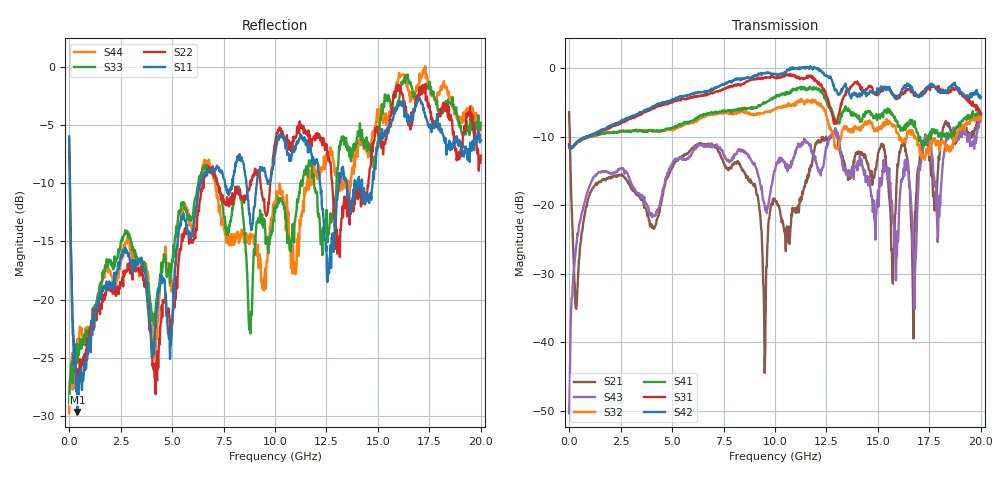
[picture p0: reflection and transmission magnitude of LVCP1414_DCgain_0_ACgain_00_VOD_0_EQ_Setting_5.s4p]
!Agilent Technologies,N5230A,MY46400459,A.07.50.48
!Agilent N5230A: A.07.50.48
!Date: Tuesday, April 17, 2012 18:35:00
!Correction: S11(Full 4 Port(1,2,3,4))
!S12(Full 4 Port(1,2,3,4))
!S13(Full 4 Port(1,2,3,4))
!S14(Full 4 Port(1,2,3,4))
!S21(Full 4 Port(1,2,3,4))
!S22(Full 4 Port(1,2,3,4))
!S23(Full 4 Port(1,2,3,4))
!S24(Full 4 Port(1,2,3,4))
!S31(Full 4 Port(1,2,3,4))
!S32(Full 4 Port(1,2,3,4))
!S33(Full 4 Port(1,2,3,4))
!S34(Full 4 Port(1,2,3,4))
!S41(Full 4 Port(1,2,3,4))
!S42(Full 4 Port(1,2,3,4))
!S43(Full 4 Port(1,2,3,4))
!S44(Full 4 Port(1,2,3,4))
!S4P File: Measurements: <S11,S12,S13,S14>,
!<S21,S22,S23,S24>,
!<S31,S32,S33,S34>,
!<S41,S42,S43,S44>:
# Hz S  dB  R 50
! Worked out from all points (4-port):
!   801 points, 300 kHz to 20 GHz, reference 50 ohm
!   strongest paths, dB at 300 kHz, 5 GHz, 10 GHz, 15 GHz, 20 GHz:
!     S42: -11.4, -4.5, -0.8, -3.1, -4.2
!     S31: -11.1, -5.0, -1.4, -3.9, -6.6
!     S41: -11.2, -8.6, -4.3, -7.1, -6.6
!     S32: -11.3, -9.0, -6.0, -9.0, -7.4
!     S43: -50.4, -13.9, -15.0, -17.8, -7.5
!     S21: -6.4, -14.5, -19.2, -12.4, -7.0
!   lowest |S11| = -29.7 dB at 400.3 MHz (marker M1), VSWR 1.07, Z = 53.1 + j1.45 ohm
!   |S11| at or under -10 dB: 37.44 MHz to 6.372 GHz (6.335 GHz wide, 198 % of centre); 8.612 GHz to 9.121 GHz (509.1 MHz wide, 5.74 % of centre); 12.19 GHz to 13.1 GHz (907.5 MHz wide, 7.18 % of centre)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
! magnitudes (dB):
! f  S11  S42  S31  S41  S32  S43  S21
! 300 kHz  -6.0  -11.4  -11.1  -11.2  -11.3  -50.4  -6.4
! 400.3 MHz  -29.7  -10.7  -10.7  -10.8  -10.8  -24.1  -32.5
! 6.325 GHz  -10.1  -3.5  -4.0  -6.9  -7.4  -11.2  -10.9
! 9.5 GHz  -9.0  -0.6  -1.4  -5.1  -6.3  -20.1  -44.5
! 12.88 GHz  -14.6  -2.8  -8.1  -7.4  -10.6  -9.3  -9.4
! 16.8 GHz  -3.5  -3.5  -3.8  -8.5  -9.9  -29.7  -21.0
! 20 GHz  -6.3  -4.2  -6.6  -6.6  -7.4  -7.5  -7.0
